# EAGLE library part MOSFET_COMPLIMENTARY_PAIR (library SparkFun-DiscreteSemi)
Complementary pair enhancement mode MOSFET A P and N channel MOSFET in a single package. Rated to breakdown at 20V Link to datasheet SparkFun Products: ZX Distance and Gesture Sensor
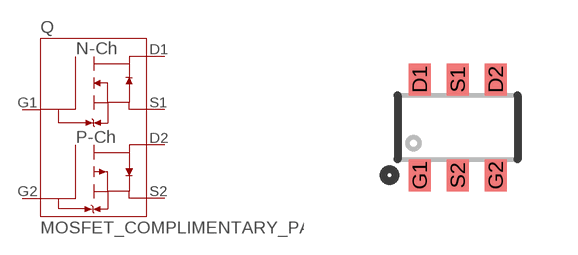
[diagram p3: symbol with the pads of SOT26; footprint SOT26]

Designator prefix Q

## MOSFET_COMPLIMENTARY_PAIR-DMC2700UDM (PROD_ID: TRANS-11993)  [SOT26]
D1  D1
D2  D2
G1  G1
G2  G2
S1  S1
S2  S2

## Footprint SOT26 (pad centres in mm)
Footprint for SOT-26 part DMP2240UDM
smd 0.55 x 0.8: D1 -0.95,1.2; D2 0.95,1.2; G1 -0.95,-1.2; G2 0.95,-1.2; S1 0,1.2; S2 0,-1.2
